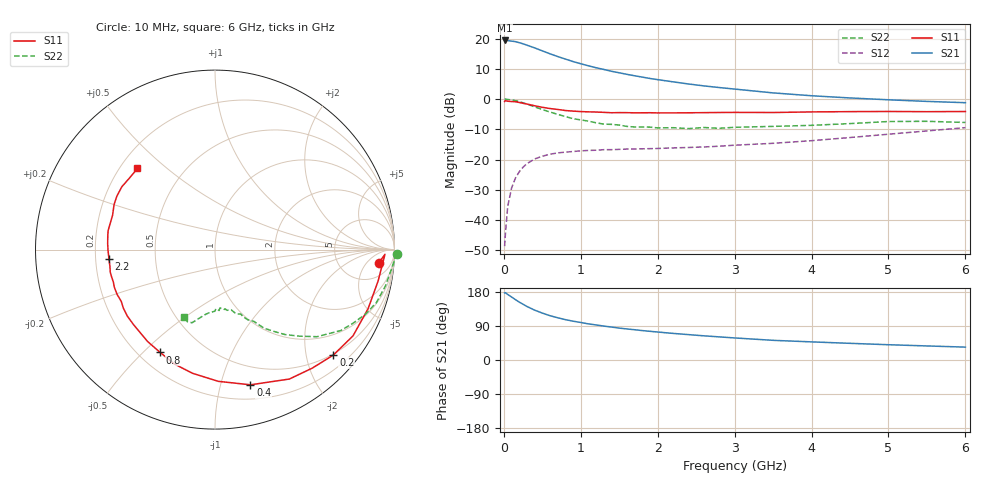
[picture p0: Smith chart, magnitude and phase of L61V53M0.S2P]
!  INFINEON TECHNOLOGIES Small Signal Semiconductors
! BFR380L3 , Si-NPN RF-Transistor in TSLP-3-1
!  Vce=1.5 V,  Ic=3 mA
! Common Emitter S-Parameters:  07. March 2005
#  GHz  S  MA  R  50
! f  S11  S21  S12  S22
! GHz  Mag  Ang  Mag  Ang  Mag  Ang  Mag  Ang
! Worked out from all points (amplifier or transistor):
!   36 points, 10 MHz to 6 GHz, reference 50 ohm
!   highest |S21| = 19.4 dB at 10 MHz (marker M1)
!   |S21| within 3 dB of that: start of sweep to 455.2 MHz
!   unconditionally stable (mu >= 1): 2.636 GHz to 4.759 GHz
!   at 250 MHz: K = 0.12, MSG = 20.4 dB, |S12| = -22.5 dB
!   at 1.4 GHz: K = 0.65, MSG = 13.0 dB, |S12| = -16.7 dB
!   at 6 GHz: K = 0.94, MSG = 4.1 dB, |S12| = -9.4 dB
!   S11 on the Smith chart (normalised r, x): 10 MHz: 12, -11; 200 MHz: 0.48, -2.55; 400 MHz: 0.32, -1.24; 800 MHz: 0.28, -0.56; 2.2 GHz: 0.26, -0.04; 6 GHz: 0.27, +0.40
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0.01  0.9158 -4.6  9.369 177.0  0.0037 88.4  1.014 -1.3
0.02  0.9474 -1.6  9.315 177.6  0.0058 89.4  1.004 -2.6
0.05  0.9255 -10.9  9.331 173.0  0.0167 85.4  0.9899 -6.2
0.1  0.9143 -21.1  9.144 166.3  0.0337 78.4  0.9703 -12.2
0.15  0.9068 -32.0  8.953 159.4  0.0493 72.4  0.9462 -18.2
0.2  0.8832 -41.7  8.613 152.8  0.0628 68.2  0.9127 -23.2
0.3  0.8318 -60.1  7.834 141.3  0.0858 59.1  0.8326 -32.8
0.4  0.7788 -75.3  7.06 131.6  0.1026 51.8  0.7473 -40.5
0.5  0.7341 -88.6  6.305 123.8  0.1138 46.9  0.6738 -45.7
0.6  0.7004 -100.3  5.636 116.9  0.123 42.4  0.6134 -50.5
0.7  0.6764 -109.6  5.078 111.5  0.1291 39.9  0.5609 -54.3
0.8  0.6493 -118.1  4.609 106.5  0.1331 37.4  0.5162 -58.0
0.9  0.6351 -126.2  4.195 102.4  0.1362 35.9  0.4759 -60.3
1.1  0.6171 -137.3  3.566 95.3  0.1419 34.2  0.4329 -64.8
1.5  0.5998 -155.4  2.733 84.2  0.1478 33.3  0.3736 -72.1
1.9  0.597 -167.9  2.202 75.7  0.152 34.8  0.3451 -78.8
2.2  0.5931 -175.1  1.936 70.2  0.1563 37.3  0.3375 -81.1
2.8  0.6023 172.7  1.558 61.0  0.1667 43.2  0.3301 -89.3
3.5  0.6019 161.4  1.271 51.9  0.1862 49.2  0.3548 -95.8
4.5  0.6225 151.5  1.048 44.0  0.2321 57.3  0.3948 -103.3
5.5  0.6212 140.2  0.919 37.1  0.2985 60.3  0.4306 -110.9
6  0.6252 133.7  0.875 34.0  0.3381 59.8  0.4121 -115.2
